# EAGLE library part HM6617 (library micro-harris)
MICROCONTROLLER/MEMORY DEVICE
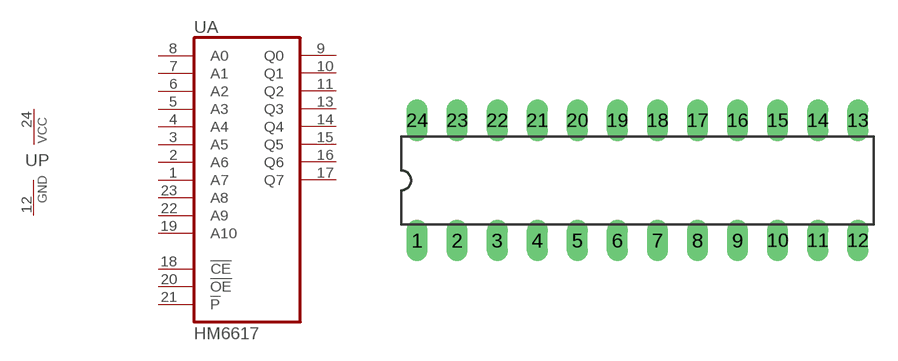
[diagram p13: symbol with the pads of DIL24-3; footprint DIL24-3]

Designator prefix U; gates A=HM6617 P=PWRN

## HM6617 (OC_FARNELL: unknown; OC_NEWARK: unknown)  [DIL24-3]
1  A:A7  in
2  A:A6  in
3  A:A5  in
4  A:A4  in
5  A:A3  in
6  A:A2  in
7  A:A1  in
8  A:A0  in
9  A:Q0  hiz
10  A:Q1  hiz
11  A:Q2  hiz
12  P:GND  pwr
13  A:Q3  hiz
14  A:Q4  hiz
15  A:Q5  hiz
16  A:Q6  hiz
17  A:Q7  hiz
18  A:!CE  in
19  A:A10  in
20  A:!OE  in
21  A:!P  in
22  A:A9  in
23  A:A8  in
24  P:VCC  pwr

## Footprint DIL24-3 (pad centres in mm)
Dual In Line Package 0.3 inch
drill 0.813 long: 1 -13.97,-3.81; 2 -11.43,-3.81; 3 -8.89,-3.81; 4 -6.35,-3.81; 5 -3.81,-3.81; 6 -1.27,-3.81; 7 1.27,-3.81; 8 3.81,-3.81; 9 6.35,-3.81; 10 8.89,-3.81; 11 11.43,-3.81; 12 13.97,-3.81; 13 13.97,3.81; 14 11.43,3.81; 15 8.89,3.81; 16 6.35,3.81; 17 3.81,3.81; 18 1.27,3.81; 19 -1.27,3.81; 20 -3.81,3.81; 21 -6.35,3.81; 22 -8.89,3.81; 23 -11.43,3.81; 24 -13.97,3.81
